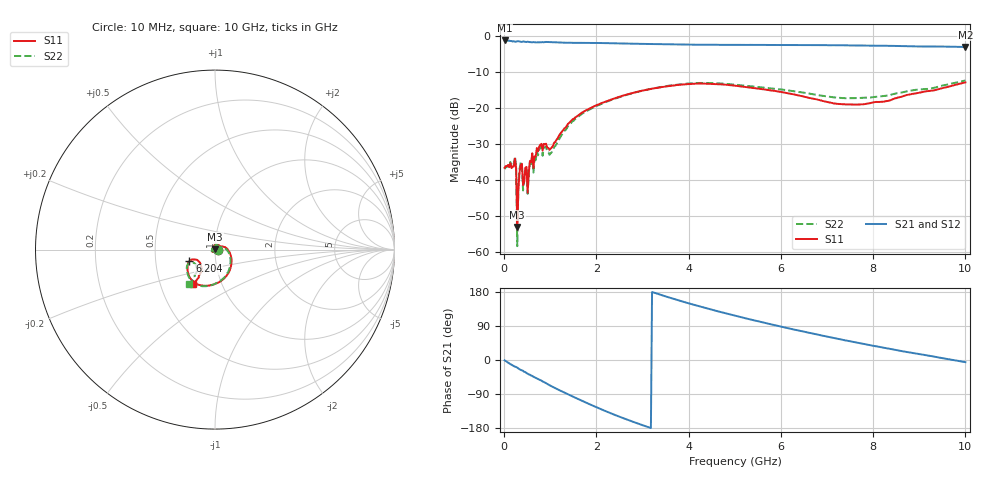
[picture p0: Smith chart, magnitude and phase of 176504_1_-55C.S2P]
!  2-Port S-parameters saved by WinCal
! VAR MeasName=S-Parameters (CALIBRATED_DATA) read from VNA (N5242A)
! VAR MeasDate=2017-11-2 17:07:09
! VAR NAME=176504_1_-55C
! VAR FILENAME=176504_1_-55C.S2P
! VAR DATE=2017-11-2 17:07:09
! VAR PHYS_PORTS=2,3
# Hz S DB R 50
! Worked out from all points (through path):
!   401 points, 10 MHz to 10 GHz, reference 50 ohm
!   highest |S21| = -1.29 dB at 10 MHz (marker M1); lowest = -3.1 dB at 10 GHz (marker M2)
!   lowest |S11| = -53.1 dB at 284.7 MHz (marker M3), VSWR 1.00, Z = 50.1 + j0.196 ohm
!   |S11| at or under -10 dB: start of sweep to end of sweep
!   |S22| runs from -58.5 to -12.4 dB; largest |S21 - S12| = 0.0065
!   S11 on the Smith chart (normalised r, x): 10 MHz: 1.03, -0.00; 6.204 GHz: 0.74, -0.10; 10 GHz: 0.73, -0.29
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1e7  -36.67 -3.1  -1.29 -0.9  -1.29 -0.9  -37.05 -4.2
2.098e8  -36.33 -121.5  -1.51 -16.0  -1.51 -16.0  -35.65 -122.6
2.34775e8  -34.11 -151.4  -1.62 -17.7  -1.62 -17.7  -33.51 -150.5
2.84725e8  -53.13 62.7  -1.49 -20.2  -1.49 -20.2  -58.47 104.8
3.34675e8  -37.83 -145.8  -1.58 -24.6  -1.58 -24.6  -36.87 -143.5
3.5965e8  -35.91 -169.7  -1.65 -26.3  -1.65 -26.2  -35.22 -165.9
3.84625e8  -35.56 157.5  -1.70 -27.4  -1.70 -27.4  -35.30 162.5
4.34575e8  -40.59 -175.1  -1.62 -31.2  -1.62 -31.2  -39.63 -165.1
4.5955e8  -36.69 108.3  -1.67 -31.9  -1.67 -31.9  -37.55 113.9
7.5925e8  -30.82 75.2  -1.83 -51.6  -1.83 -51.6  -31.70 77.3
9.84025e8  -31.73 29.8  -1.73 -66.6  -1.73 -66.6  -33.08 23.6
1.433575e9  -23.88 7.6  -1.95 -93.3  -1.94 -93.3  -24.47 4.7
1.683325e9  -21.37 -12.6  -1.94 -107.4  -1.94 -107.3  -21.70 -15.7
2.482525e9  -16.99 -54.4  -2.11 -148.9  -2.10 -148.8  -17.11 -56.6
3.35665e9  -14.38 -89.6  -2.32 173.5  -2.33 173.5  -14.32 -90.8
4.180825e9  -13.28 -116.8  -2.46 143.4  -2.48 143.5  -13.12 -115.8
5.005e9  -13.85 -136.7  -2.51 116.9  -2.51 117.1  -13.58 -134.7
6.2038e9  -16.09 -155.6  -2.55 82.6  -2.54 82.6  -15.23 -151.4
6.678325e9  -17.43 -155.9  -2.55 70.1  -2.57 70.2  -16.22 -152.1
7.55245e9  -19.11 -141.4  -2.67 48.1  -2.68 48.2  -17.34 -142.9
8.35165e9  -17.97 -126.0  -2.76 29.6  -2.80 29.8  -16.51 -131.2
1e10  -12.94 -122.7  -3.11 -5.6  -3.12 -5.3  -12.41 -127.9
